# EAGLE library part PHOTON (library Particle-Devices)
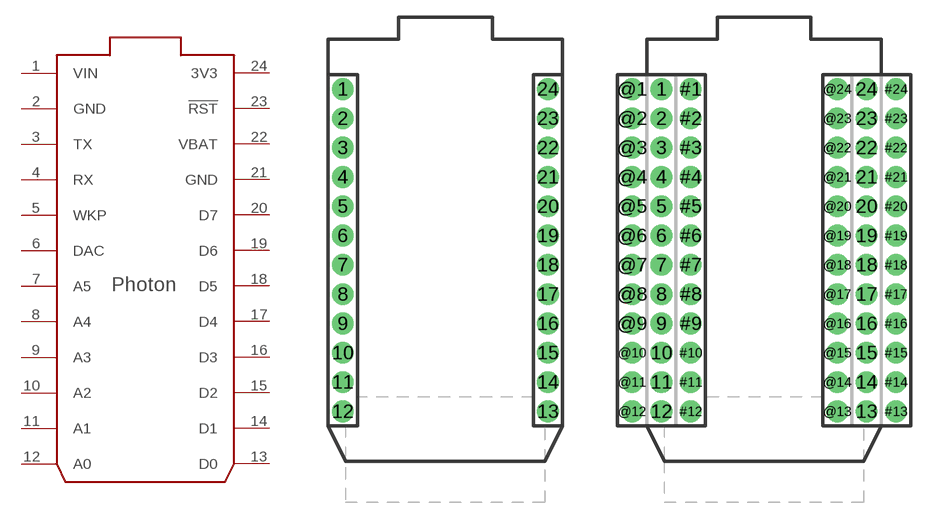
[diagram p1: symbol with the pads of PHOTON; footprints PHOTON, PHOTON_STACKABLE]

Designator prefix -

## PHOTON_WITH_HEADERS  [PHOTON]
1  VIN  pwr
2  GND  pwr
3  TX
4  RX
5  WKP
6  DAC
7  A5
8  A4
9  A3
10  A2
11  A1
12  A0
13  D0
14  D1
15  D2
16  D3
17  D4
18  D5
19  D6
20  D7
21  GND  pwr
22  VBAT  pwr
23  !RST
24  3V3  pwr

## PHOTON_WITH_STACKABLE_HEADERS  [PHOTON_STACKABLE]
1  VIN  pwr
2  GND  pwr
3  TX
4  RX
5  WKP
6  DAC
7  A5
8  A4
9  A3
10  A2
11  A1
12  A0
13  D0
14  D1
15  D2
16  D3
17  D4
18  D5
19  D6
20  D7
21  GND  pwr
22  VBAT  pwr
23  !RST
24  3V3  pwr
#1  VIN  pwr
#2  GND  pwr
#3  TX
#4  RX
#5  WKP
#6  DAC
#7  A5
#8  A4
#9  A3
#10  A2
#11  A1
#12  A0
#13  D0
#14  D1
#15  D2
#16  D3
#17  D4
#18  D5
#19  D6
#20  D7
#21  GND  pwr
#22  VBAT  pwr
#23  !RST
#24  3V3  pwr
@1  VIN  pwr
@2  GND  pwr
@3  TX
@4  RX
@5  WKP
@6  DAC
@7  A5
@8  A4
@9  A3
@10  A2
@11  A1
@12  A0
@13  D0
@14  D1
@15  D2
@16  D3
@17  D4
@18  D5
@19  D6
@20  D7
@21  GND  pwr
@22  VBAT  pwr
@23  !RST
@24  3V3  pwr

## Footprint PHOTON (pad centres in mm)
drill 1.016 pad 1.88: 1 1.27,32.258; 2 1.27,29.718; 3 1.27,27.178; 4 1.27,24.638; 5 1.27,22.098; 6 1.27,19.558; 7 1.27,17.018; 8 1.27,14.478; 9 1.27,11.938; 10 1.27,9.398; 11 1.27,6.858; 12 1.27,4.318; 13 19.05,4.318; 14 19.05,6.858; 15 19.05,9.398; 16 19.05,11.938; 17 19.05,14.478; 18 19.05,17.018; 19 19.05,19.558; 20 19.05,22.098; 21 19.05,24.638; 22 19.05,27.178; 23 19.05,29.718; 24 19.05,32.258

## Footprint PHOTON_STACKABLE (pad centres in mm)
drill 1.016 pad 1.88: 1 1.27,32.258; 2 1.27,29.718; 3 1.27,27.178; 4 1.27,24.638; 5 1.27,22.098; 6 1.27,19.558; 7 1.27,17.018; 8 1.27,14.478; 9 1.27,11.938; 10 1.27,9.398; 11 1.27,6.858; 12 1.27,4.318; 13 19.05,4.318; 14 19.05,6.858; 15 19.05,9.398; 16 19.05,11.938; 17 19.05,14.478; 18 19.05,17.018; 19 19.05,19.558; 20 19.05,22.098; 21 19.05,24.638; 22 19.05,27.178; 23 19.05,29.718; 24 19.05,32.258; #1 3.81,32.258; #2 3.81,29.718; #3 3.81,27.178; #4 3.81,24.638; #5 3.81,22.098; #6 3.81,19.558; #7 3.81,17.018; #8 3.81,14.478; #9 3.81,11.938; #10 3.81,9.398; #11 3.81,6.858; #12 3.81,4.318; #13 21.59,4.318; #14 21.59,6.858; #15 21.59,9.398; #16 21.59,11.938; #17 21.59,14.478; #18 21.59,17.018; #19 21.59,19.558; #20 21.59,22.098; #21 21.59,24.638; #22 21.59,27.178; #23 21.59,29.718; #24 21.59,32.258; @1 -1.27,32.258; @2 -1.27,29.718; @3 -1.27,27.178; @4 -1.27,24.638; @5 -1.27,22.098; @6 -1.27,19.558; @7 -1.27,17.018; @8 -1.27,14.478; @9 -1.27,11.938; @10 -1.27,9.398; @11 -1.27,6.858; @12 -1.27,4.318; @13 16.51,4.318; @14 16.51,6.858; @15 16.51,9.398; @16 16.51,11.938; @17 16.51,14.478; @18 16.51,17.018; @19 16.51,19.558; @20 16.51,22.098; @21 16.51,24.638; @22 16.51,27.178; @23 16.51,29.718; @24 16.51,32.258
